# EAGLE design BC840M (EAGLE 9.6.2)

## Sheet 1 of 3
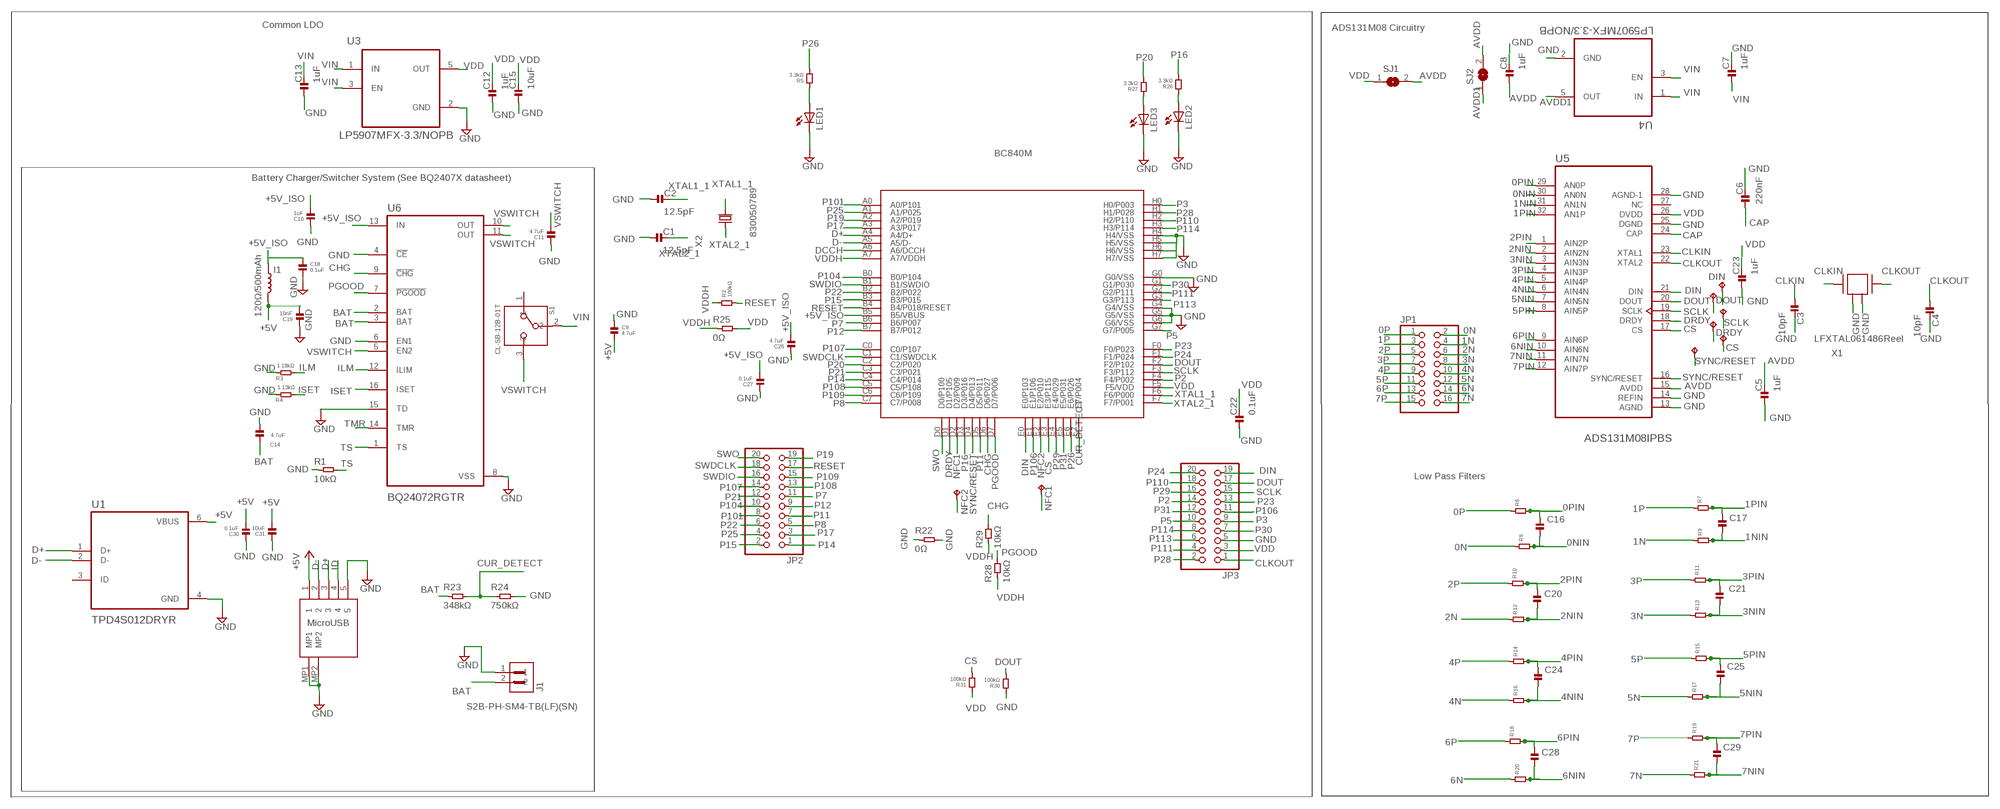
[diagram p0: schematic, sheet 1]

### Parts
C1  12.5pF  CAPACITOR.0201  [0201]
C2  12.5pF  CAPACITOR.0201  [0201]
C3  10pF  CAPACITOR.0201  [0201]
C4  10pF  CAPACITOR.0201  [0201]
C5  1uF  CAPACITOR.0201  [0201]
C6  220nF  CAPACITOR.0201  [0201]
C7  1uF  CAPACITOR.0201  [0201]
C8  1uF  CAPACITOR.0201  [0201]
C9  4.7uF  CAPACITOR.0201  [0201]
C10  1uF  CAPACITOR.0201  [0201]
C11  4.7uF  CAPACITOR.0201  [0201]
C12  1uF  CAPACITOR.0201  [0201]
C13  1uF  CAPACITOR.0201  [0201]
C14  4.7uF  CAPACITOR.0201  [0201]
C15  10uF  CAPACITOR.0402  [0402]
C16  100pF  CAPACITOR.0603  [0603]
C17  100pF  CAPACITOR.0603  [0603]
C18  0.1uF  CAPACITOR.0201  [0201]
C19  10nF  CAPACITOR.0201  [0201]
C20  100pF  CAPACITOR.0603  [0603]
C21  100pF  CAPACITOR.0603  [0603]
C22  0.1uF  CAPACITOR.0201  [0201]
C23  1uF  CAPACITOR.0201  [0201]
C24  100pF  CAPACITOR.0603  [0603]
C25  100pF  CAPACITOR.0603  [0603]
C26  4.7uF  CAPACITOR.0201  [0201]
C27  0.1uF  CAPACITOR.0201  [0201]
C28  100pF  CAPACITOR.0603  [0603]
C29  100pF  CAPACITOR.0603  [0603]
C30  0.1uF  CAPACITOR.0201  [0201]
C31  10uF  CAPACITOR.0402  [0402]
CS  TPTP07R  [TP07R]
DIN  TPTP07R  [TP07R]
DOUT  TPTP07R  [TP07R]
DRDY  TPTP07R  [TP07R]
I1  120Ω/500mAh  12NH-0402  [0402_COILCRAFT]
J1  S2B-PH-SM4-TB(LF)(SN)  [JST_S2B-PH-SM4-TB(LF)(SN)]
JP1  PINHD-2X8SMT  [2X08_SMT]
JP2  PINHD-2X10SMT  [2X10_SMT]
JP3  PINHD-2X10SMT  [2X10_SMT]
LED1  LEDCHIPLED_0603  [CHIPLED_0603]
LED2  LEDCHIPLED_0603  [CHIPLED_0603]
LED3  LEDCHIPLED_0603  [CHIPLED_0603]
NFC1  TPTP14SQ  [TP14SQ]
NFC2  TPTP14SQ  [TP14SQ]
R1  10kΩ  RESISTOR.0201  [0201]
R2  100kΩ  RESISTOR.0201  [0201]
R3  1.18kΩ  RESISTOR.0603  [0603]
R4  1.13kΩ  RESISTOR.0603  [0603]
R5  3.3kΩ  RESISTOR.0201  [0201]
R6  1MOhm  RESISTOR.0603  [0603]
R7  1MOhm  RESISTOR.0603  [0603]
R8  1MOhm  RESISTOR.0603  [0603]
R9  1MOhm  RESISTOR.0603  [0603]
R10  1MOhm  RESISTOR.0603  [0603]
R11  1MOhm  RESISTOR.0603  [0603]
R12  1MOhm  RESISTOR.0603  [0603]
R13  1MOhm  RESISTOR.0603  [0603]
R14  1MOhm  RESISTOR.0603  [0603]
R15  1MOhm  RESISTOR.0603  [0603]
R16  1MOhm  RESISTOR.0603  [0603]
R17  1MOhm  RESISTOR.0603  [0603]
R18  1MOhm  RESISTOR.0603  [0603]
R19  1MOhm  RESISTOR.0603  [0603]
R20  1MOhm  RESISTOR.0603  [0603]
R21  1MOhm  RESISTOR.0603  [0603]
R22  0Ω  RESISTOR.0805  [0805]
R23  348kΩ  RESISTOR.0603  [0603]
R24  750kΩ  RESISTOR.0603  [0603]
R25  0Ω  RESISTOR.0805  [0805]
R26  3.3kΩ  RESISTOR.0201  [0201]
R27  3.3kΩ  RESISTOR.0201  [0201]
R28  10kΩ  RESISTOR.0402  [0402]
R29  10kΩ  RESISTOR.0402  [0402]
R30  100kΩ  RESISTOR.0402  [0402]
R31  100kΩ  RESISTOR.0402  [0402]
S1  CL-SB-12B-01T  [CL-SB-12B]
SCLK  TPTP07R  [TP07R]
SJ1  SJ  [SJ]
SJ2  SJ  [SJ]
SYNC  TPTP07R  [TP07R]
U1  TPD4S012DRYR  [PSON50P145X100X60-6N]
U2  BC840M  [BC840M]
U3  LP5907MFX-3.3/NOPB  [SOT95P280X145-5N]
U4  LP5907MFX-3.3/NOPB  [SOT95P280X145-5N]
U5  ADS131M08IPBS  [QFP50P700X700X120-32N]
U6  BQ24072RGTR  [QFN50P300X300X100-17N]
U7  DX4R005JJ2R1800  [DX4R005JJ2R1800]
X1  ABM3B-8.000MHZ-B2-T  [ABM3B-8.000MHZ-B2-T]
X2  FC-12M  [FC-12M]

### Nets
0N: JP1.2 R8.1
0NIN: C16.2 R8.2 U5.30(AN0N)
0P: JP1.1 R6.1
0PIN: C16.1 R6.2 U5.29(AN0P)
1N: JP1.4 R9.1
1NIN: C17.2 R9.2 U5.31(AN1N)
1P: JP1.3 R7.1
1PIN: C17.1 R7.2 U5.32(AN1P)
2N: JP1.6 R12.1
2NIN: C20.2 R12.2 U5.2(AIN2N)
2P: JP1.5 R10.1
2PIN: C20.1 R10.2 U5.1(AIN2P)
3N: JP1.8 R13.1
3NIN: C21.2 R13.2 U5.3(AIN3N)
3P: JP1.7 R11.1
3PIN: C21.1 R11.2 U5.4(AIN3P)
4N: JP1.10 R16.1
4NIN: C24.2 R16.2 U5.6(AIN4N)
4P: JP1.9 R14.1
4PIN: C24.1 R14.2 U5.5(AIN4P)
5N: JP1.12 R17.1
5NIN: C25.2 R17.2 U5.7(AIN5N)
5P: JP1.11 R15.1
5PIN: C25.1 R15.2 U5.8(AIN5P)
6N: JP1.14 R20.1
6NIN: C28.2 R20.2 U5.10(AIN6N)
6P: JP1.13 R18.1
6PIN: C28.1 R18.2 U5.9(AIN6P)
7N: JP1.16 R21.1
7NIN: C29.2 R21.2 U5.11(AIN7N)
7P: JP1.15 R19.1
7PIN: C29.1 R19.2 U5.12(AIN7P)
+5V: C9.2 C19.2 C30.2 C31.2 I1.P$2 U1.6(VBUS) U7.1
+5V_ISO: C10.2 C18.1 C26.2 C27.2 I1.P$1 U2.B5(B5/VBUS) U6.13(IN)
AVDD: C5.2 C8.1 SJ1.2 SJ2.2 U5.15(AVDD)
AVDD1: SJ2.1 U4.5(OUT)
BAT: C14.2 J1.2 R23.1 U6.2(BAT) U6.3(BAT)
CAP: C6.1 U5.24(CAP)
CHG: R29.2 U2.D6(D6/P027) U6.9(!CHG)
CLKIN: C3.1 U5.23(XTAL1) X1.1
CLKOUT: C4.1 JP3.1 U5.22(XTAL2) X1.3
CS: CS.TP R31.1 U2.E3(E3/P115) U5.17(CS)
CUR_DETECT: R23.2 R24.1 U2.E7(E7/P004)
D+: U1.1(D+) U2.A4(A4/D+) U7.3
D-: U1.2(D-) U2.A5(A5/D-) U7.2
DCCH: U2.A6(A6/DCCH)
DIN: DIN.TP JP3.19 U2.E0(E0/P103) U5.21(DIN)
DOUT: DOUT.TP JP3.17 R30.1 U2.F2(F2/P102) U5.20(DOUT)
DRDY: DRDY.TP U2.D1(D1/P105) U5.18(DRDY)
GND: C1.1 C2.1 C3.2 C4.2 C5.1 C6.2 C7.2 C8.2 C9.1 C10.1 C11.1 C12.1 C13.1 C14.1 C15.1 C18.2 C19.1 C22.1 C23.1 C26.1 C27.1 C30.1 C31.1 J1.1 JP3.5 LED1.C LED2.C LED3.C R1.1 R3.1 R4.1 R22.1 R22.2 R24.2 R30.2 U1.4(GND) U2.G0(G0/VSS) U2.G4(G4/VSS) U2.G5(G5/VSS) U2.G6(G6/VSS) U2.H4(H4/VSS) U2.H5(H5/VSS) U2.H6(H6/VSS) U2.H7(H7/VSS) U3.2(GND) U4.2(GND) U5.13(AGND) U5.14(REFIN) U5.25(DGND) U5.28(AGND-1) U6.4(!CE) U6.6(EN1) U6.8(VSS) U6.15(TD) U7.5 U7.MP1 U7.MP2 X1.2 X1.4
ID: U7.4
ILM: R3.2 U6.12(ILIM)
ISET: R4.2 U6.16(ISET)
LED1: LED1.A R5.2
LED2: LED2.A R26.2
LED3: LED3.A R27.2
NFC1: NFC2.TP U2.D2(D2/P009)
NFC2: NFC1.TP U2.E2(E2/P010)
P2: JP3.14 U2.F4(F4/P002)
P3: JP3.9 U2.H0(H0/P003)
P5: JP3.10 U2.G7(G7/P005)
P7: JP2.11 U2.B6(B6/P007)
P8: JP2.5 U2.C7(C7/P008)
P11: JP2.7 U2.D5(D5/P011)
P12: JP2.9 U2.B7(B7/P012)
P14: JP2.1 U2.C4(C4/P014)
P15: JP2.2 U2.B3(B3/P015)
P16: R26.1 U2.D3(D3/P016)
P17: JP2.3 U2.A3(A3/P017)
P19: JP2.19 U2.A2(A2/P019)
P20: R27.1 U2.C2(C2/P020)
P21: JP2.12 U2.C3(C3/P021)
P22: JP2.6 U2.B2(B2/P022)
P23: JP3.13 U2.F0(F0/P023)
P24: JP3.20 U2.F1(F1/P024)
P25: JP2.4 U2.A1(A1/P025)
P26: R5.1 U2.E6(E6/P026)
P28: JP3.2 U2.H1(H1/P028)
P29: JP3.16 U2.E4(E4/P029)
P30: JP3.7 U2.G1(G1/P030)
P31: JP3.12 U2.E5(E5/P031)
P101: JP2.8 U2.A0(A0/P101)
P104: JP2.10 U2.B0(B0/P104)
P106: JP3.11 U2.E1(E1/P106)
P107: JP2.14 U2.C0(C0/P107)
P108: JP2.13 U2.C5(C5/P108)
P109: JP2.15 U2.C6(C6/P109)
P110: JP3.18 U2.H2(H2/P110)
P111: JP3.4 U2.G2(G2/P111)
P113: JP3.6 U2.G3(G3/P113)
P114: JP3.8 U2.H3(H3/P114)
PGOOD: R28.2 U2.D7(D7/P006) U6.7(!PGOOD)
RESET: JP2.17 R2.1 U2.B4(B4/P018/RESET)
SCLK: JP3.15 SCLK.TP U2.F3(F3/P112) U5.19(SCLK)
SWDCLK: JP2.18 U2.C1(C1/SWDCLK)
SWDIO: JP2.16 U2.B1(B1/SWDIO)
SWO: JP2.20 U2.D0(D0/P100)
SYNC/RESET: SYNC.TP U2.D4(D4/P013) U5.16(SYNC/RESET)
TMR: U6.14(TMR)
TS: R1.2 U6.1(TS)
VDD: C12.2 C15.2 C22.2 C23.2 JP3.3 R25.2 R31.2 SJ1.1 U2.F5(F5/VDD) U3.5(OUT) U5.26(DVDD)
VDDH: R2.2 R25.1 R28.1 R29.1 U2.A7(A7/VDDH)
VIN: C7.1 C13.2 S1.2 U3.1(IN) U3.3(EN) U4.1(IN) U4.3(EN)
VSWITCH: C11.2 S1.3 U6.5(EN2) U6.10(OUT) U6.11(OUT)
XTAL1_1: C2.2 U2.F6(F6/P000) X2.2
XTAL2_1: C1.2 U2.F7(F7/P001) X2.1
Unconnected: S1.1 U1.3(ID) U5.27(NC)

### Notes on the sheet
- Common LDO
- ADS131M08 Circuitry
- BC840M
- Battery Charger/Switcher System (See BQ2407X datasheet)
- 830050789
- LFXTAL061486Reel
- Low Pass Filters
- MicroUSB

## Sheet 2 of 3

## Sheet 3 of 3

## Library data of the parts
C1-C31 = standardparts:CAPACITOR
CS DIN DOUT DRDY NFC1 NFC2 SCLK SYNC = testpad:TP: Test pad
I1 = spkfncoils:12NH; MOUSER_PART: 994-0402HP-12NXGLU; PROD_ID: NDUC-15271; VALUE: 12nH
J1 = S2B-PH-SM4-TB_LF__SN_:S2B-PH-SM4-TB(LF)(SN): CONN HEADER PH SIDE 2POS 2MM SMD Check prices; AVAILABILITY: In Stock; DESCRIPTION: Connector Header Surface Mount, Right Angle 2 position 0.079 (2.00mm); MF: JST Sales; MP: S2B-PH-SM4-TB (LF)(SN); PACKAGE: None; PRICE: None
JP1 = pinhead+:PINHD-2X8: PIN HEADER
JP2 JP3 = pinhead+:PINHD-2X10: PIN HEADER
LED1-LED3 = adafruit:LED: LED
R1 R2 R4-R31 = standardparts:RESISTOR
R3 = standardparts:RESISTOR; SPICEPREFIX: R
S1 = CL-SB-12B-01T:CL-SB-12B-01T: Check prices; AVAILABILITY: In Stock; DESCRIPTION: Slide Switch SPDT Surface Mount; MF: Nidec Copal; MP: CL-SB-12B-01T; PACKAGE: None; PRICE: None
SJ1 SJ2 = jumper:SJ: SMD solder JUMPER
U1 = TPD4S012DRYR:TPD4S012DRYR: Check prices; AVAILABILITY: In Stock; DESCRIPTION: 4-channel USB ESD solution with power clamp 6-SON -40 to 85; MF: Texas Instruments; MP: TPD4S012DRYR; PACKAGE: USON-6 Texas Instruments; PRICE: None; PURCHASE-URL: https://pricing.snapeda.com/search/part/TPD4S012DRYR/?ref=eda
U2 = BC840M:BC840M: Check prices; AVAILABILITY: In Stock; DESCRIPTION: 802.15.4, Bluetooth Bluetooth v5.0, Thread, Zigbee® Transceiver Module 2.4GHz PCB Trace Surface Mount; MF: Fanstel Corp.; MP: BC840M; PACKAGE: None; PRICE: None; PURCHASE-URL: https://pricing.snapeda.com/search/part/BC840M/?ref=eda
U3 U4 = LP5907MFX-3.3_NOPB:LP5907MFX-3.3/NOPB: IC REG LINEAR 3.3V 250MA SOT23; AVAILABILITY: Unavailable; DESCRIPTION: Linear Voltage Regulator IC 1 Output 250mA SOT-23-5; MF: Texas Instruments; MP: LP5907MFX-3.3/NOPB; PACKAGE: SOT-23 Texas Instruments; PRICE: None
U5 = ADS131M08IPBS:ADS131M08IPBS: None Check prices; AVAILABILITY: Warning; DESCRIPTION: 24-bit 32-kSPS 8-channelsimultaneous-sampling delta-sigma ADC 32-TQFP -40 to 125; MF: Texas Instruments; MP: ADS131M08IPBS; PACKAGE: TQFP-32 Texas Instruments; PRICE: None; PURCHASE-URL: https://pricing.snapeda.com/search/part/ADS131M08IPBS/?ref=eda
U6 = BQ24072RGTR:BQ24072RGTR: Check prices; AVAILABILITY: In Stock; DESCRIPTION: Standalone 1-cell 1.5-A linear charger, Power Path, 4.2-V VBAT and VOUT=VBAT + 225mV 16-VQFN -40 to 85; MF: Texas Instruments; MP: BQ24072RGTR; PACKAGE: VQFN-16 Texas Instruments; PRICE: None; PURCHASE-URL: https://pricing.snapeda.com/search/part/BQ24072RGTR/?ref=eda
U7 = DX4R005JJ2R1800:DX4R005JJ2R1800: Check prices; AVAILABILITY: In Stock; DESCRIPTION: USB - micro B USB 2.0 Receptacle Connector 5 Position Surface Mount, Right Angle; Through Hole; MF: JAE Electronics; MP: DX4R005JJ2R1800; PACKAGE: None; PRICE: None
X1 = Crystals_Oscillators:ABM3B-8.000MHZ-B2-T: CRYSTAL 8.0000MHZ 18PF SMD Manufacturer's datasheet; CREATED_BY: PCBLayout.com; DIGIKEY_PART_NUMBER: 535-9720-2-ND; MANUFACTURER: Abracon LLC; MPN: ABM3B-8.000MHZ-B2-T; PACKAGE: SMD 4
X2 = crystal:FC-12M: kHz RANGE CRYSTAL UNIT

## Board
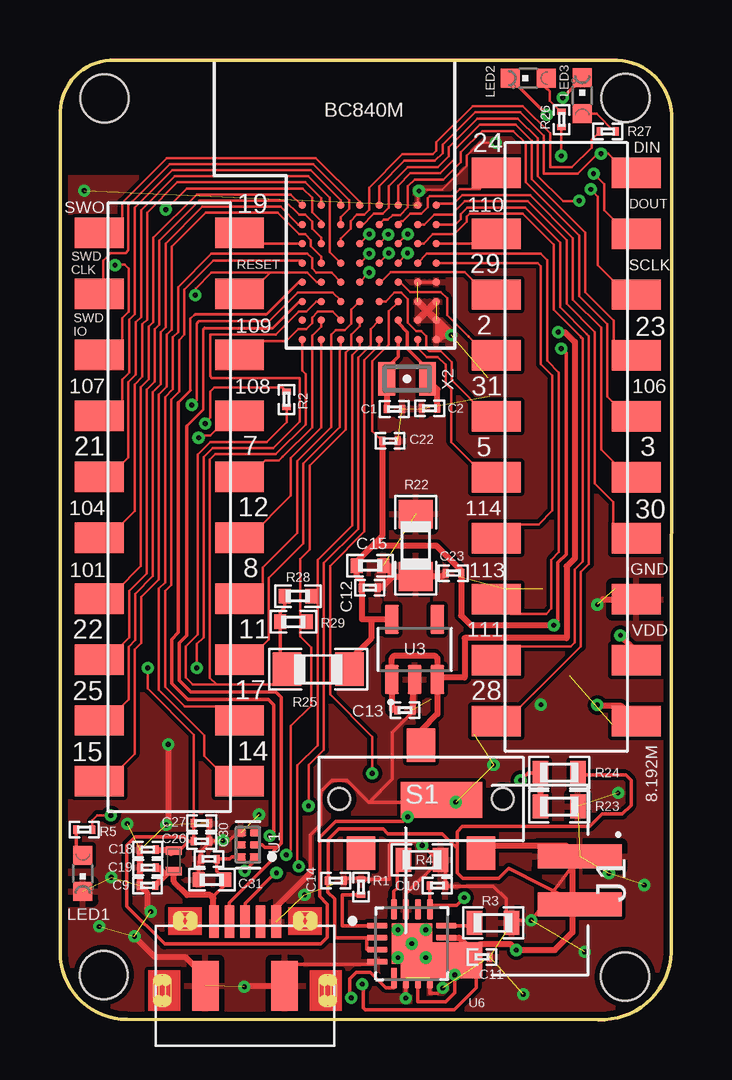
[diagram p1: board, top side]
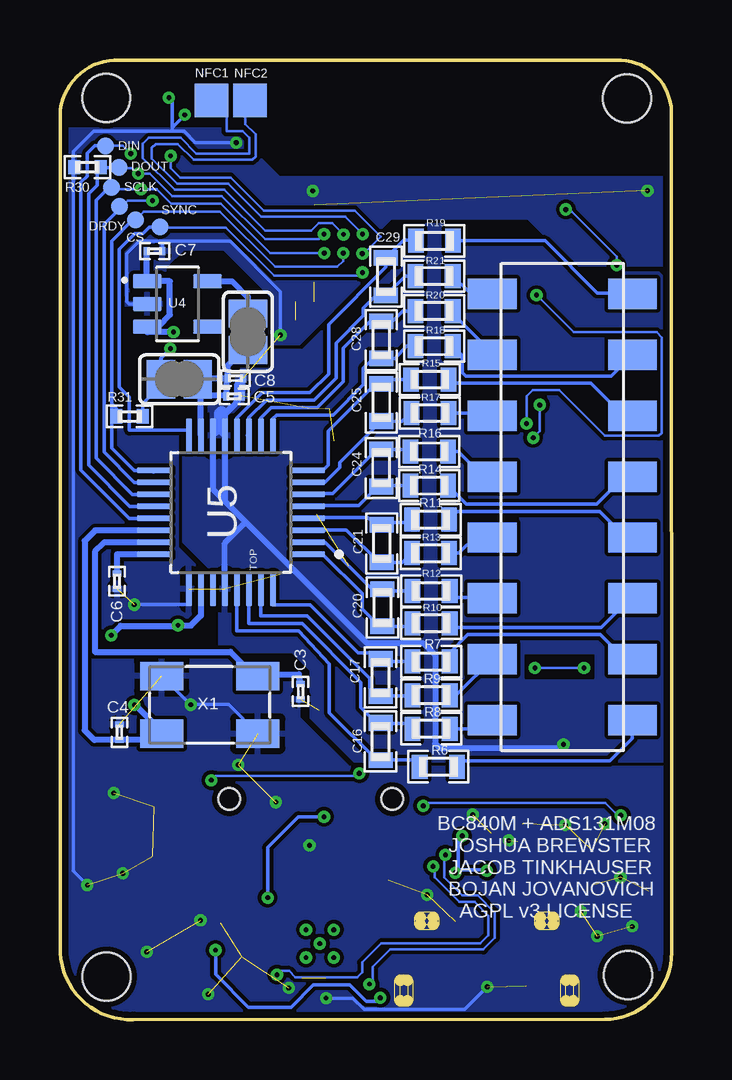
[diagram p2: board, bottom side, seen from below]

Size 25.49 x 40 mm. Coordinates in mm from the lower left corner, seen from the top.
Outline: 0,2.8 0.01,37.84 arc-90 2.3,40 23,40 arc-90 25.49,37.71 25.48,2.79 arc-90 22.43,0 2.79,0 arc-90 0,2.8
Copper layers (1*16): Top 0.035mm / dielectric 1.5mm / Bottom 0.035mm
Design rules "default *": minimum track width 4mil, minimum drill 0.2mm, track to track 6mil, track to pad 6mil, pad to pad 6mil, via to via 6mil, smd to smd 6mil, copper to edge 10mil, drill to drill 6mil, minimum pad ring 6mil, minimum via ring 6mil, stop-mask expansion 4mil, vias tented up to drill 0mil, thermal gap 10mil
Holes 2 mm at 1.86,38.4 23.56,38.42 1.82,1.86 23.54,1.79

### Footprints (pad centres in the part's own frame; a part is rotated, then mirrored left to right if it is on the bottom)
0201 = smd 0.25 x 0.35: 1 -0.325,0; 2 0.325,0
0402 = smd 0.5 x 0.6: 1 -0.55,0; 2 0.55,0
0603 = smd 0.65 x 1: 1 -0.775,0; 2 0.775,0
TP07R = smd 0.7 x 0.7: TP 0,0
0402_COILCRAFT = smd 0.356 x 0.66: P$1 -0.432,0; P$2 0.432,0
JST_S2B-PH-SM4-TB(LF)(SN) = smd 1 x 3.5: 1 1,0; 2 -1,0 | smd 1.5 x 3.4: P1 3.35,5.75; P2 -3.35,5.75
2X08_SMT = smd 1.27 x 2.032: 1 -8.89,-2.921; 2 -8.89,2.921; 3 -6.35,-2.921; 4 -6.35,2.921; 5 -3.81,-2.921; 6 -3.81,2.921; 7 -1.27,-2.921; 8 -1.27,2.921; 9 1.27,-2.921; 10 1.27,2.921; 11 3.81,-2.921; 12 3.81,2.921; 13 6.35,-2.921; 14 6.35,2.921; 15 8.89,-2.921; 16 8.89,2.921
2X10_SMT = smd 1.27 x 2.032: 1 -11.43,-2.921; 2 -11.43,2.921; 3 -8.89,-2.921; 4 -8.89,2.921; 5 -6.35,-2.921; 6 -6.35,2.921; 7 -3.81,-2.921; 8 -3.81,2.921; 9 -1.27,-2.921; 10 -1.27,2.921; 11 1.27,-2.921; 12 1.27,2.921; 13 3.81,-2.921; 14 3.81,2.921; 15 6.35,-2.921; 16 6.35,2.921; 17 8.89,-2.921; 18 8.89,2.921; 19 11.43,-2.921; 20 11.43,2.921
CHIPLED_0603 = smd 0.8 x 0.8: A 0,-0.75; C 0,0.75
TP14SQ = smd 1.4 x 1.4: TP 0,0
0805 = smd 1.2 x 1.4: 1 -1.3,0; 2 1.3,0
CL-SB-12B = smd 1.2 x 1.4: 1 -2.5,-2.25; 2 0,2.25; 3 2.5,-2.25 | hole 0.9: 3.4,0; -3.4,0
SJ = smd 1.168 x 1.6: 1 -0.762,0; 2 0.762,0
PSON50P145X100X60-6N = smd 0.42 x 0.3: 1 -0.29,0.5 | smd 0.41 x 0.3: 2 -0.295,0; 3 -0.295,-0.5; 4 0.295,-0.5; 5 0.295,0; 6 0.295,0.5
BC840M = smd 0.305 x 0.305: A0 0.66,5.966; A1 0.66,5.153; A2 0.66,4.366; A3 0.66,3.553; A4 0.66,2.765; A5 0.66,1.953; A6 0.66,1.165; A7 0.66,0.352; B0 1.448,5.966; B1 1.448,5.153; B2 1.448,4.366; B3 1.448,3.553; B4 1.448,2.765; B5 1.448,1.953; B6 1.448,1.165; B7 1.448,0.352; C0 2.261,5.966; C1 2.261,5.153; C2 2.261,4.366; C3 2.261,3.553; C4 2.261,2.765; C5 2.261,1.953; C6 2.261,1.165; C7 2.261,0.352; D0 3.048,5.966; D1 3.048,5.153; D2 3.048,4.366; D3 3.048,3.553; D4 3.048,2.765; D5 3.048,1.953; D6 3.048,1.165; D7 3.048,0.352; E0 3.861,5.966; E1 3.861,5.153; E2 3.861,4.366; E3 3.861,3.553; E4 3.861,2.765; E5 3.861,1.953; E6 3.861,1.165; E7 3.861,0.352; F0 4.648,5.966; F1 4.648,5.153; F2 4.648,4.366; F3 4.648,3.553; F4 4.648,2.765; F5 4.648,1.953; F6 4.648,1.165; F7 4.648,0.352; G0 5.461,5.966; G1 5.461,5.153; G2 5.461,4.366; G3 5.461,3.553; G4 5.461,2.765; G5 5.461,1.953; G6 5.461,1.165; G7 5.461,0.352; H0 6.248,5.966; H1 6.248,5.153; H2 6.248,4.366; H3 6.248,3.553; H4 6.248,2.765; H5 6.248,1.953; H6 6.248,1.165; H7 6.248,0.352
SOT95P280X145-5N = smd 1.21 x 0.59: 1 -1.255,0.95; 2 -1.255,0; 3 -1.255,-0.95; 4 1.255,-0.95; 5 1.255,0.95
QFP50P700X700X120-32N = smd 1.44 x 0.26: 1 -3.195,1.75; 2 -3.195,1.25; 3 -3.195,0.75; 4 -3.195,0.25; 5 -3.195,-0.25; 6 -3.195,-0.75; 7 -3.195,-1.25; 8 -3.195,-1.75; 17 3.195,-1.75; 18 3.195,-1.25; 19 3.195,-0.75; 20 3.195,-0.25; 21 3.195,0.25; 22 3.195,0.75; 23 3.195,1.25; 24 3.195,1.75 | smd 0.26 x 1.44: 9 -1.75,-3.195; 10 -1.25,-3.195; 11 -0.75,-3.195; 12 -0.25,-3.195; 13 0.25,-3.195; 14 0.75,-3.195; 15 1.25,-3.195; 16 1.75,-3.195; 25 1.75,3.195; 26 1.25,3.195; 27 0.75,3.195; 28 0.25,3.195; 29 -0.25,3.195; 30 -0.75,3.195; 31 -1.25,3.195; 32 -1.75,3.195
QFN50P300X300X100-17N = smd 0.86 x 0.26: 1 -1.435,0.75; 2 -1.435,0.25; 3 -1.435,-0.25; 4 -1.435,-0.75; 9 1.435,-0.75; 10 1.435,-0.25; 11 1.435,0.25; 12 1.435,0.75 | smd 0.26 x 0.86: 5 -0.75,-1.435; 6 -0.25,-1.435; 7 0.25,-1.435; 8 0.75,-1.435; 13 0.75,1.435; 14 0.25,1.435; 15 -0.25,1.435; 16 -0.75,1.435 | smd 1.68 x 1.68: 17 0,0 | drill 0.2 pad 0.4: 18 0,0; 19 -0.58,0.58; 20 0.58,0.58; 21 -0.58,-0.58; 22 0.58,-0.58
DX4R005JJ2R1800 = smd 1.35 x 0.4: 1 1.525,1.3; 2 1.525,0.65; 3 1.525,0; 4 1.525,-0.65; 5 1.525,-1.3 | smd 2.1 x 1.1: MP1 -1.15,1.65; MP2 -1.15,-1.65
ABM3B-8.000MHZ-B2-T = smd 1.8 x 1.2: 1 -2,-1.2; 2 2,-1.2; 3 2,1.2; 4 -2,1.2
FC-12M = smd 0.7 x 1.4: 1 -0.85,0; 2 0.85,0

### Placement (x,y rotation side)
C1  13.93,25.45 180 top
C2  15.4,25.48 0 top
C3  15.46,13.68 270 bottom
C4  23.01,11.98 90 bottom
C5  18.23,25.98 180 bottom
C6  23.11,18.27 270 bottom
C7  21.54,32.03 0 bottom
C8  18.18,26.74 0 bottom
C9  3.64,5.59 0 top
C10  15.72,5.58 180 top
C11  17.58,2.61 180 top
C12  12.91,18.01 180 top
C13  14.38,12.9 180 top
C14  11.49,5.8 180 top
C15  12.92,18.93 180 top
C16  12.13,11.59 90 bottom
C17  12.13,14.26 270 bottom
C18  3.66,7.08 180 top
C19  3.66,6.34 0 top
C20  12.05,17.17 90 bottom
C21  12.08,19.85 270 bottom
C22  13.75,24.12 180 top
C23  16.39,18.61 0 top
C24  12.11,23 90 bottom
C25  12.1,25.73 270 bottom
C26  5.9,7.43 180 top
C27  5.9,8.19 180 top
C28  12.1,28.33 90 bottom
C29  11.91,30.97 270 bottom
C30  6.21,6.7 0 top
C31  6.33,5.83 0 top
CS  22.34,33.34 0 bottom
DIN  23.59,36.42 0 bottom
DOUT  23.04,35.52 0 bottom
DRDY  23.01,33.9 0 bottom
I1  4.74,6.61 270 top
J1  21.65,5.81 90 top
JP1  4.56,21.37 90 bottom
JP2  4.55,21.36 90 top
JP3  21.09,23.87 90 top
LED1  0.95,6.09 180 top
LED2  19.5,39.25 90 top
LED3  21.76,38.52 0 top
NFC1  19.18,38.32 0 bottom
NFC2  17.57,38.32 0 bottom
R1  12.55,5.53 270 top
R2  9.44,25.85 270 top
R3  18.04,4.03 180 top
R4  15.08,6.66 180 top
R5  1.01,7.92 180 top
R6  9.73,10.54 180 bottom
R7  10.03,14.92 180 bottom
R8  10.03,12.13 180 bottom
R9  10.03,13.52 180 bottom
R10  10.03,16.52 180 bottom
R11  10.05,20.84 180 bottom
R12  10.03,17.87 180 bottom
R13  10.05,19.44 180 bottom
R14  10.1,22.26 180 bottom
R15  10.08,26.68 180 bottom
R16  10.1,23.68 180 bottom
R17  10.07,25.29 180 bottom
R18  9.9,28.07 180 bottom
R19  9.89,32.46 180 bottom
R20  9.9,29.54 180 bottom
R21  9.9,31 180 bottom
R22  14.82,19.77 90 top
R23  20.8,10.29 180 top
R24  20.8,8.88 0 top
R25  10.76,14.6 0 top
R26  20.9,37.52 90 top
R27  22.82,37.02 0 top
R28  9.92,17.65 0 top
R29  9.72,16.58 0 top
R30  24.35,35.53 180 bottom
R31  22.59,25.14 0 bottom
S1  15.04,9.19 0 top
SCLK  23.35,34.7 0 bottom
SJ1  20.52,26.7 0 bottom
SJ2  17.66,28.67 270 bottom
SYNC  21.32,33.04 0 bottom
U1  7.83,7.28 180 top
U2  9.44,27.99 0 top
U3  14.78,15.43 90 top
U4  20.6,29.83 0 bottom
U5  18.37,21.14 180 bottom
U6  14.66,3.17 0 top
U7  7.71,2.56 90 top
X1  19.25,13.12 180 bottom
X2  14.47,26.72 0 top

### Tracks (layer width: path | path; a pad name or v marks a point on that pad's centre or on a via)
0N
  Bottom 0.152: R8.1 7.83,12.13 JP1.2
0NIN
  Bottom 0.152: U5.30 17.62,16.5 15.41,16.5 12.95,14.05 12.95,13 12.31,12.37 C16.2 12.12,12.35 11.03,12.35 R8.2
0P
  Bottom 0.152: R6.1 8.95,10.78 2.59,10.78 1.64,11.73 JP1.1
0PIN
  Bottom 0.152: U5.29 18.12,16.2 15.54,16.2 14.26,14.82 14.26,12.79 12.29,10.82 C16.1 10.78,10.82 R6.2
1N
  Bottom 0.152: R9.1 9.19,13.59 8.91,13.59 JP1.4
1NIN
  Bottom 0.152: U5.31 17.12,16.83 15.19,16.83 12.58,14.23 12.58,13.81 12.26,13.48 C17.2 12.13,13.5 10.83,13.5 R9.2
1P
  Bottom 0.152: R7.1 9.25,15.29 8.49,16.05 2.98,16.05 1.95,15.02 JP1.3
1PIN
  Bottom 0.152: U5.32 16.62,17.28 15.06,17.28 13.06,15.28 12.38,15.28 C17.1 12.02,14.92 R7.2
2N
  Bottom 0.152: R12.1 8.98,17.6 7.52,17.6 JP1.6
2NIN
  Bottom 0.152: R12.2 11.97,17.87 C20.2 12.5,17.94 14.45,19.89 U5.2 | U5.2 | U5.2
2P
  Bottom 0.152: R10.1 9.08,16.35 2.94,16.35 1.73,17.56 JP1.5
2PIN
  Bottom 0.152: U5.1 14.53,19.39 12.9,17.76 12.9,17.12 12.18,16.39 C20.1 10.93,16.39 R10.2
3N
  Bottom 0.152: R13.1 8.87,19.44 8.17,20.14 7.52,20.14 JP1.8
3NIN
  Bottom 0.152: R13.2 11.22,19.05 12.06,19.05 C21.2 12.21,19.07 13.55,20.42 15.15,20.42 U5.3
3P
  Bottom 0.152: R11.1 8.94,21.18 3,21.18 1.92,20.1 JP1.7
3PIN
  Bottom 0.152: U5.4 15.13,20.93 12.67,20.93 12.36,20.62 C21.1 11.99,20.71 10.95,20.71 R11.2
4N
  Bottom 0.152: JP1.10 7.85,22.64 8.9,23.68 R16.1
4NIN
  Bottom 0.152: U5.6 15.13,21.93 14.12,21.93 12.29,23.77 C24.2 12.1,23.76 10.96,23.76 R16.2
4P
  Bottom 0.152: R14.1 8.55,21.49 3.12,21.49 1.97,22.64 JP1.9
4PIN
  Bottom 0.152: U5.5 15.13,21.43 13.04,21.43 12.25,22.22 C24.1 12.11,22.26 R14.2
5N
  Bottom 0.152: R17.1 7.59,25.29 JP1.12
5NIN
  Bottom 0.152: U5.7 15.15,22.42 14.43,22.42 13.83,23.02 13.83,23.22 C25.2 11.25,24.94 10.9,25.29 R17.2
5P
  Bottom 0.152: R15.1 9.15,26.53 3.37,26.53 2.02,25.18 JP1.11
5PIN
  Bottom 0.152: U5.8 14.54,22.89 14.31,23.12 14.31,24.54 12.35,26.5 C25.1 11.92,26.68 R15.2
6N
  Bottom 0.152: R20.1 9.08,29.49 9.08,29.39 7.49,27.81 7.49,27.73 JP1.14
6NIN
  Bottom 0.152: U5.10 17.12,25.07 16.68,25.51 14.77,25.51 13.68,26.6 13.68,27.99 12.56,29.11 C28.2 11.63,29.11 11.21,29.52 10.69,29.52 R20.2
6P
  Bottom 0.152: R18.1 8.72,27.67 8.72,26.97 8.59,26.83 2.52,26.83 JP1.13
6PIN
  Bottom 0.152: U5.9 16.62,25.05 16.46,25.2 14.11,25.2 12.85,26.46 12.85,27.15 12.44,27.56 C28.1 11.55,27.56 11.03,28.07 R18.2
7N
  Bottom 0.152: R21.1 8.43,30.3 7.52,30.3 JP1.16
7NIN
  Bottom 0.152: U5.11 17.62,25.09 16.88,25.83 14.9,25.83 13.98,26.74 13.98,28.21 12.85,29.35 12.85,29.67 12.32,30.19 C29.2 11.11,31 R21.2
  Bottom 0.254: U5.11
7P
  Bottom 0.152: R19.1 5.28,32.46 3.11,30.29 1.65,30.29 1.64,30.28 JP1.15
7PIN
  Bottom 0.152: U5.12 18.12,25.07 17.06,26.13 15.08,26.13 14.29,26.92 14.29,28.98 11.91,31.36 C29.1 11.16,32.5 10.7,32.5 R19.2
+5V
  Top 0.102: 6.43,4.11 U7.1
  Top 0.152: 4.73,6.17 I1.P$2 4.69,6.24 | 4.04,6.29 C19.2 | U1.6 7.15,6.78 7.07,6.7 C30.2 6.54,6.17 C31.2 6.88,5.62 6.39,5.13 6.39,5.06
  Top 0.254: U7.1 6.39,4.1 6.39,5.06 6.26,5.19 5.29,5.19 4.75,5.74 I1.P$2 | 4.73,6.17 4.55,6.17 C9.2 4.28,5.9 4.28,6.17 4.11,6.34 C19.2
+5V_ISO  (via drill 0.2)
  Top 0.102: U2.B5 10.69,29.94 10.26,29.51 9.95,29.51 8.99,28.55 6.27,28.55 6.26,28.54 6.26,26.82 6.33,26.75 9.98,26.75 9.98,24.93 8.88,23.82 6.36,23.82 5.99,23.45 5.99,15.94 5.7,15.65 v5.7,14.66 | v3.66,14.66 3.66,13.8 5.58,11.88 C27.2 | I1.P$1
  Top 0.152: v14.49,8.45 14.31,8.27 11.49,8.27 10.81,7.6 10.81,5.14 11.15,4.81 11.15,3.44 10.86,3.15 4.36,3.15 2.78,4.73 2.78,7.26 3.13,7.61 5.19,7.61 5.36,7.43 C26.2 | C18.1 | v16.84,5.08 16.53,4.77 15.41,4.77 U6.13 C10.2 | C26.2 5.37,7.43 4.99,7.05 I1.P$1 | C27.2 C26.2
  Top 0.254: C18.1 4.49,7.08 4.63,6.93 I1.P$1
  Bottom 0.102: v5.7,14.66 v3.66,14.66
  Bottom 0.152: v14.49,8.45 15.56,8.45 16.84,7.17 v16.84,5.08
AVDD
  Bottom 0.254: U5.15 19.62,26.02 18.6,26.02 C5.2 18.56,26.68 C8.1 | C8.1 18.5,26.74 | C8.1 18.5,27.25 17.85,27.91 SJ2.2 | SJ1.2 19.71,26.74 C8.1
AVDD1
  Bottom 0.254: U4.5 18.32,30.78 17.66,30.12 SJ2.1
BAT
  Top 0.152: J1.2 18.7,6.31 18.28,5.89 16.77,5.89 16.54,6.12 16.54,7.13 | R23.1 21.68,10.19 23.57,10.19 23.8,9.96 23.8,8.93 23.43,8.57 22.59,8.57 22.08,8.06 16.77,8.06 16.54,7.83 16.54,7.13 | 16.54,7.13 15.92,7.75 13.66,7.75 13.46,7.95 11.61,7.95 11.17,7.51 C14.2 11.17,5.31 11.45,5.03 11.45,3.42 12.77,3.42 | U6.3 13.21,2.93 12.77,2.93 12.77,3.42 | U6.2 12.77,3.42
CAP
  Bottom 0.254: U5.24 23.11,19.39 C6.1
CHG  (via drill 0.2)
  Top 0.102: U2.D6 12.48,28.9 12.13,28.55 12.13,28.02 11.91,27.8 11.91,24.59 10.41,23.09 10.41,19.6 10.01,19.2 10.01,16.63 | v9.43,6.87 9.62,7.07 9.62,12.23 10.46,13.07 10.46,15.52 10.01,15.98 10.01,16.63 | R29.2 10.22,16.63 10.01,16.63
  Top 0.152: U6.9 16.67,2.42 17.34,1.75 17.34,1.33 16.42,0.41 12.71,0.41 12.63,0.5 12.63,1.45 v12.6,1.48
  Bottom 0.102: v9.43,6.87 9.48,6.82 9.48,5.93 8.72,5.17 8.09,5.17 7.37,4.46 7.37,3.4 7.85,2.92 11.73,2.92 12.46,2.19 12.46,1.61 v12.6,1.48
CLKIN
  Bottom 0.254: U5.23 23.64,19.89 24.03,19.51 24.03,15.33 18.39,15.33 17.38,14.32 X1.1 17.17,14.39 15.53,14.39 C3.1
CLKOUT  (via drill 0.2)
  Top 0.254: v22.39,13.11 22.4,13.1 23.36,13.1 JP3.1
  Bottom 0.254: X1.3 21.65,11.92 | U5.22 24.02,20.39 24.46,19.95 24.46,12.06 24.06,11.65 C4.1 21.51,11.65 X1.3 | v22.39,13.11 22.35,13.11 21.25,12.01 X1.3
CS  (via drill 0.2 pad 0.15)
  Top 0.102: U2.E3 13.3,31.55 v13.69,31.95 | v13.69,31.95
  Bottom 0.102: v13.69,31.95 13.69,31.61 13.93,31.38 16.53,31.38 18.83,33.68 22,33.68 CS.TP
  Bottom 0.152: U5.17 22.4,22.89 23.34,23.82 23.34,25.67 | 23.34,25.67 23.34,32.46 22.45,33.34 CS.TP | R31.1 23.14,25.48 23.34,25.67
  Bottom 0.254: U5.17 21.58,22.87
CUR_DETECT  (via drill 0.2)
  Top 0.102: U2.E7 13.3,28.11 12.68,27.49 12.68,20.34 11.25,18.92 11.25,13.55 13.02,11.79 v13.02,10.26
  Top 0.152: v19.19,9.98 19.5,10.29 R23.2
  Top 0.254: R24.1 R23.2
  Bottom 0.102: v13.02,10.26 13.12,10.16 19.01,10.16 v19.19,9.98
D+  (via drill 0.2)
  Top 0.102: U2.A4 9.95,30.75 | 5.61,29.39 5.43,29.21 5.43,26.23
  Top 0.127: 9.95,30.75 8.59,29.39 5.61,29.39 | 4.94,25.73 5.43,26.23
  Top 0.152: U7.3 7.71,4.85 8.98,6.12 v9.02,6.12 | v8.73,7.66 8.9,7.83 8.9,13.12 8.67,13.35 5.32,13.35 4.66,14.01 4.66,15.85 4.94,16.13 4.94,25.73 | U1.1 8.12,6.61 v7.71,6.2
  Bottom 0.152: v8.73,7.66 8.9,7.49 8.9,6.24 v9.02,6.12 8.9,6.23 7.74,6.23 v7.71,6.2
D-
  Top 0.102: U2.A5 9.97,29.94 | 6.02,28.83 5.97,28.78 5.97,25.42
  Top 0.127: 9.97,29.94 8.87,28.83 6.02,28.83 | 5.97,25.42 5.29,24.75
  Top 0.152: U7.2 7.06,4.87 8.91,6.72 8.91,7.03 9.04,7.17 | 9.04,7.17 9.22,7.35 9.22,7.43 9.22,13.03 9.22,13.42 8.98,13.66 5.45,13.66 4.96,14.14 4.96,15.69 5.29,16.02 5.29,24.75 | 9.04,7.17 8.54,7.17 8.43,7.28 U1.2
DIN  (via drill 0.2)
  Top 0.102: U2.E0 13.3,34.74 14.35,35.8 15.61,35.8 15.94,36.12 15.94,36.47 17.29,37.82 19.18,37.82 20.17,36.84 20.17,35.27 21.58,35.27 22.41,36.1 v22.54,36.1 22.55,36.11 22.84,36.11 23.65,35.3 JP3.19
  Bottom 0.102: v22.54,36.1 22.87,36.42 DIN.TP
  Bottom 0.152: U5.21 22.61,20.89 24.62,22.9 24.62,34.9 24.35,35.17 24.35,36.12 24.05,36.42 DIN.TP
DOUT  (via drill 0.2, 0.2 pad 0.15)
  Top 0.102: U2.F2 14.31,32.58 14.32,32.58 v14.49,32.75 | v22.23,35.26 22.24,35.26 22.68,34.82 22.68,33.74 23.66,32.76 JP3.17
  Bottom 0.102: v14.49,32.75 14.7,32.53 16.93,32.53 18.74,34.34 20.82,34.34 21.74,35.26 v22.23,35.26 22.47,35.5 23.02,35.5 DOUT.TP
  Bottom 0.152: U5.20 22.58,21.39 24.3,23.11 24.3,34.43 23.94,34.78 23.94,35.3 23.73,35.52 | 23.73,35.52 DOUT.TP | R30.1 23.78,35.52 23.73,35.52
DRDY  (via drill 0.2)
  Top 0.102: U2.D1 12.54,33.08 12.57,33.08 13.07,33.59 13.44,33.59 13.7,33.85 13.7,34.74 14.5,35.54 15.74,35.54 16.19,36 16.19,36.36 17.4,37.56 19.08,37.56 19.91,36.73 19.91,35.17 20.97,34.11 21.6,34.11 v21.64,34.14
  Bottom 0.102: v21.64,34.14 22.66,34.14 22.91,33.9 DRDY.TP
  Bottom 0.152: U5.18 22.39,22.39 23.65,23.66 23.65,33.16 22.96,33.85 DRDY.TP
GND  (via drill 0.2)  (36 unrouted)
  Top 0.102: U2.G0 14.9,34.37 15.01,34.48 | 15.01,34.48 15.12,34.59 15.94,34.59 16.95,35.61 16.95,36.02 17.49,36.56 v18.15,36.56 | v14.96,34.54 15.01,34.49 15.01,34.48
  Top 0.152: U6.8 15.41,1.1 15.73,1.1 v15.95,1.32 | U7.5 9.01,4.7 | C13.1 14.7,12.82 13.85,11.96 13.85,10.02 12.88,9.06 | LED3.C 21.76,39.24 v20.95,38.43 | v20.29,37.71 LED2.C | 13.23,2.37 U6.4 13.11,2.3 9.9,2.3 9.36,1.76 U7.MP2 | U6.15 14.41,5.24 15.83,6.66 R4.1 | R4.1 16.05,6.47 C10.1 16.07,5.56 18.06,5.56 18.59,5.03 18.59,4.25 R3.1 18.93,4.13 v19.63,4.13 19.68,4.18 J1.1 | R1.1 12.5,5.9 11.92,5.9 C14.1 | R1.1 13.72,5.85 13.72,7.29 13.86,7.43 14.93,7.43 v15.09,7.26 15.11,7.26 15.71,6.66 R4.1 | R1.1 | U2.G4 U2.H4 | U6.6 14.41,0.9 v14.4,0.89 | 10.43,6.12 10.43,7.71 10.86,8.14 10.86,9.52 11.32,9.97 11.97,9.97 12.88,9.06 | 12.88,9.06 v16.49,9.06 | C31.1 5.78,6.59 C30.1 5.89,7.03 6.32,7.46 v6.79,7.46 7.06,7.46 7.38,7.79 U1.4 | 6.42,7.43 C26.1 C27.1
  Top 0.254: U7.MP1 6.06,1.78 5.23,2.6 3.96,2.6 v3.1,3.47 | U3.2 14.7,14.1 14.7,13.87 | 14.7,13.87 C13.1 | 14.7,13.87 | 9.01,4.7 10.43,6.12 | v4.51,11.48 4.51,8.29 4.43,8.21 v4.43,8.12 | v7.68,1.37 7.73,1.41 U7.MP2 | C18.2 C19.1 3.32,6.32 C9.1 3.64,5.28 3.64,4.65 v3.79,4.5 | 13.87,18.47 13.4,18.01 C12.1 | 13.87,18.47 13.75,18.47 13.75,18.86 13.68,18.93 C15.1 | 13.87,18.47 R22.1 15.92,18.47 C23.1 | v22.39,17.29 22.62,17.52 JP3.5
  Top 0.305: U2.G5 U2.H6 | U2.G6 U2.H5 | U2.H6 16.3,28.55 v16.3,28.53 | v16.3,28.53 v16.31,28.53 15.93,28.53 15.79,28.38 | v16.3,28.53 | 15.79,28.38 15.75,28.34 U2.H7 | U2.H6 15.79,29.05 15.79,28.38
  Bottom 0.102: C8.2 17.84,26.73
  Bottom 0.152: U4.2 22.6,29.83 22.71,29.94 22.71,31.94 22.19,32.45 21.2,32.45 | v18.15,36.56 19.85,36.56 20.32,37.03 20.81,37.03 | 24.93,35.57 24.93,36.19 24.09,37.03 20.81,37.03 | 24.93,35.57 24.93,6.19 v24.35,5.61 | v20.29,37.71 v20.29,37.7 20.61,37.38 20.81,37.19 | v20.95,38.43 20.81,38.29 20.81,37.19 | 20.81,37.19 20.81,37.03 | 21.2,32.45 21.22,32.43 C7.2 | v16.3,28.53 16.3,30.35 18.4,32.45 21.2,32.45 | 18.7,25.3 18.77,25.22 | 18.56,25.33 18.7,25.19 18.7,25.3 | 18.7,25.45 18.7,25.3 | R30.2 24.93,35.57 | U5.25 20.12,17.29 v22.39,17.29 | X1.4 18.46,13.13 v20.04,13.13 20.06,13.13 X1.2 | v14.4,0.89 13.28,0.89 12.82,0.43 8.62,0.43 v7.68,1.37
  Bottom 0.254: 18.32,25.53 18.36,25.53 18.56,25.33 | 18.77,25.22 18.77,24.5 U5.13 | 18.7,25.45 18.81,25.45 18.95,25.3 18.95,24.5 U5.14 19.12,22.11 18.62,21.61 | 18.15,25.69 18.1,25.74 18.1,26.49 C8.2 17.91,26.68 C5.1 18.15,25.74 18.15,25.69 | 18.62,21.61 17.74,20.74 | 17.74,20.74 12.7,15.7 10.36,15.7 9.86,15.19 9.86,11.51 9.67,11.33 4.66,11.33 v4.51,11.48 | U5.28 18.62,19.86 17.74,20.74 | U5.13 18.62,21.61 | 18.15,25.69 18.32,25.53 | 18.32,25.53 18.62,25.23 U5.13
  other vias: 2.13,5.93 18.06,10.62 21.87,2.82 22.87,6.09 1.01,34.55 23.25,9.44 2.8,8.17 19.31,1.05 8.29,8.54 1.64,3.88 10.19,5.2
  pour Top: 1.46,-0.28 -0.01,1.19 -0.01,35.1 16.75,35.1 16.75,36.07 17.75,37.07 25.64,37.07 25.64,1.36 24,-0.28
  pour Bottom: -0.29,30.28 0.55,31.11 4.1,31.11 6.13,33.14 11.47,33.14 12.47,32.14 12.47,30.78 15.36,27.88 16.89,27.88 16.89,30.03 18.7,31.84 20.24,31.84 20.82,31.25 20.82,28.53 20.32,28.03 20.32,19.9 18.83,18.41 18.83,15.35 15.82,15.35 15.02,14.55 15.02,12.57 13.24,10.78 -0.29,10.78
  pour Bottom: 0.04,31.44 4.01,31.44 5.97,33.41 11.71,33.41 12.68,32.44 12.68,31.03 15.52,28.19 16.67,28.19 16.67,30.14 18.65,32.13 20.36,32.13 21.12,31.36 21.12,28.38 20.6,27.87 20.6,19.67 19.09,18.16 19.09,15.37 18.76,15.04 15.97,15.04 15.53,14.6 15.53,12.57 13.47,10.5 -0.23,10.5 -0.23,1.48 1.55,-0.3 24.02,-0.3 25.69,1.37 25.69,37.12 18.39,37.12 16.36,35.1 0.04,35.1
  cutout Bottom: 3.28,15.18 3.28,14.24 6.07,14.24 6.07,15.18
ILM
  Top 0.152: U6.12 17.29,3.92 R3.2
ISET
  Top 0.152: U6.16 13.91,5.34 14.05,5.48 14.05,6.41 R4.2
LED1
  Top 0.102: R5.2
  Top 0.152: R5.2 0.68,7.11 LED1.A
LED2
  Top 0.102: LED2.A 20.25,39.24 20.25,38.85 20.4,38.69 20.4,38.31 20.86,37.84 R26.2
LED3
  Top 0.102: R27.2 23.1,37.02 22.36,37.77 LED3.A
NFC1  (via drill 0.2)
  Top 0.102: U2.D2 v12.88,32.75
  Bottom 0.102: v12.88,32.75 13.61,33.47 17.11,33.47 18.48,34.84 20.61,34.84 21.66,35.89 21.66,36.34 21.5,36.5 20.58,36.5 19.91,35.84 17.47,35.84 17.34,35.97 17.34,36.9 17.78,37.33 17.78,38.11 NFC2.TP
NFC2  (via drill 0.2)
  Top 0.102: U2.E2 v13.67,32.73
  Bottom 0.102: NFC1.TP 18.55,37.68 18.55,37.03 17.88,37.03 17.6,36.75 17.6,36.11 17.61,36.1 19.81,36.1 20.46,36.75 21.79,36.75 22.03,36.51 22.03,35.91 20.71,34.59 18.64,34.59 16.94,32.9 15.02,32.9 14.71,33.21 14.15,33.21 v13.67,32.73
P2  (1 unrouted)
  Top 0.102: U2.F4 14.17,30.75 14.59,30.33 15.86,30.33 16.13,30.07 16.13,29.37 17,28.5 | JP3.14 17.82,27.68 17.03,28.47
P3
  Top 0.102: U2.H0 15.75,34.02 16.42,34.02 16.76,34.36 19.59,34.36 21.37,32.58 21.37,30.02 22.54,28.84 22.54,23.77 23.38,22.93 23.69,22.93 JP3.9
P5
  Top 0.102: U2.G7 14.9,27.99 15.27,27.62 15.75,27.62 16.07,27.3 16.07,26.51 16.3,26.28 16.3,24.08 17.79,22.6 JP3.10
P7
  Top 0.102: U2.B6 10.88,28.89 10.5,28.51 10.5,24.69 9.29,23.48 9.12,23.31 8.54,23.31 7.87,22.63 JP2.11
P8
  Top 0.102: U2.C7 11.7,27.95 11.66,27.91 11.66,24.7 10.14,23.18 10.14,19.85 8.69,18.41 8.69,15.85 7.86,15.01 JP2.5
P11
  Top 0.102: U2.D5 12.46,29.94 12.13,29.6 12.13,29.01 11.86,28.74 11.49,28.74 11.29,28.55 11.29,24.7 9.88,23.28 9.88,20.28 8.44,18.84 8.44,18.17 7.82,17.55 JP2.7
P12
  Top 0.102: U2.B7 10.89,24.68 9.62,23.41 9.62,21.84 7.88,20.09 JP2.9
P14
  Top 0.102: U2.C4 11.32,31.13 10.69,31.13 10.5,31.31 10.5,31.74 10.31,31.93 6.31,31.93 4.92,30.54 4.92,28.65 4.71,28.44 4.71,26.28 4.38,25.95 4.38,18.23 4.12,17.97 4.12,13.74 6.02,11.84 6.02,11 7.09,9.93 JP2.1
P15
  Top 0.102: U2.B3 10.88,31.81 10.45,32.24 10.45,32.5 10.22,32.74 9.98,32.74 9.08,33.63 6.06,33.63 4.66,32.22 4.66,28.76 4.45,28.55 4.45,26.38 4.13,26.05 4.13,18.34 3.39,17.61 3.39,15.71 3.11,15.43 3.11,11.07 1.97,9.93 JP2.2
P16  (via drill 0.2, 0.2 pad 0.15)
  Top 0.102: U2.D3 12.51,31.54 v12.89,31.92 v12.89,31.93 | R26.1 20.88,37.17 v20.88,36
  Bottom 0.102: v12.89,31.93 12.84,31.93 12.13,32.64 13.21,33.73 17,33.73 18.38,35.1 20.49,35.1 20.88,35.5 v20.88,36
P17
  Top 0.102: U2.A3 10.01,31.63 6.38,31.63 5.18,30.43 5.18,28.55 4.96,28.33 4.96,26.17 4.63,25.84 4.63,18.12 4.38,17.87 4.38,13.87 5.2,13.05 6.52,13.05 7.17,12.41 7.41,12.41 JP2.3
P19
  Top 0.102: U2.A2 9.19,32.35 | 9.19,32.35 9.18,32.35 | 9.19,32.35 7.92,32.35 JP2.19
P20
  Top 0.102: U2.C2 11.7,32.55 12.11,32.96 12.11,33.29 12.37,33.55 12.67,33.55 12.88,33.77 12.88,34.69 14.27,36.07 15.53,36.07 15.68,36.23 15.68,36.57 17.19,38.07 19.29,38.07 20.42,36.94 20.42,35.53 21.33,35.53 22.15,36.35 22.15,36.67 R27.1
P21
  Top 0.102: U2.C3 11.24,32 11.24,34.25 10.34,35.15 4.78,35.15 3.38,33.75 3.38,29.29 3.16,29.07 3.16,26.88 2.85,26.58 2.85,23.43 2.05,22.63 JP2.12
P22
  Top 0.102: U2.B2 10.88,32.6 10.5,32.98 10.5,33.27 10.22,33.55 9.96,33.55 9.37,34.14 5.81,34.14 4.14,32.47 4.14,28.97 3.95,28.77 3.95,26.59 3.62,26.27 3.62,18.6 2.88,17.87 2.88,15.92 1.97,15.01 JP2.6
P23
  Top 0.102: U2.F0 14.08,34.77 14.6,35.28 15.85,35.28 16.45,35.88 16.45,36.26 17.49,37.3 18.99,37.3 19.65,36.63 19.65,35.04 21.88,32.81 21.88,30.34 23.07,29.14 23.07,28.23 23.63,27.68 JP3.13
P24
  Top 0.102: U2.F1 14.23,33.28 14.28,33.28 14.59,33.6 15.04,33.6 15.31,33.86 15.31,34.24 15.41,34.33 16.37,34.33 16.65,34.61 17.49,34.61 JP3.20
P25
  Top 0.102: U2.A1 9.94,33.14 9.19,33.88 5.93,33.88 4.4,32.35 4.4,28.86 4.2,28.66 4.2,26.49 3.87,26.16 3.87,18.48 3.14,17.75 3.14,15.82 2.86,15.54 2.86,13.35 1.98,12.47 JP2.4
P26  (via drill 0.2)
  Top 0.102: U2.E6 12.94,28.79 12.94,28.11 12.42,27.59 12.42,20.46 10.99,19.03 10.99,11.25 10.36,10.61 v10.36,8.91 | v2.12,8.51 1.55,8.51 1.33,8.3 R5.1
  Bottom 0.102: v10.36,8.91 10.24,9.03 2.77,9.03 2.25,8.51 v2.12,8.51
P28
  Top 0.102: U2.H1 15.76,33.14 16.47,33.14 16.7,33.37 16.7,33.58 16.97,33.85 19.38,33.85 20.84,32.39 20.84,29.7 21.96,28.58 22.03,28.5 22.03,18.98 21.71,18.65 21.71,15.55 18.6,12.44 JP3.2
P29
  Top 0.102: U2.E4 13.37,30.75 13.78,31.16 16.86,31.16 17.81,30.22 JP3.16
P30
  Top 0.102: U2.G1 15.18,33.14 15.59,33.55 16.45,33.55 16.45,33.69 16.86,34.11 19.48,34.11 21.11,32.49 21.11,29.85 22.29,28.67 22.29,22.34 23.05,21.58 23.05,20.7 23.68,20.06 JP3.7
P31
  Top 0.102: U2.E5 13.58,29.94 13.94,30.3 14.23,30.3 14.49,30.03 14.49,29.05 14.85,28.69 15.04,28.69 15.25,28.48 15.25,28.01 15.39,27.87 15.86,27.87 16.32,27.41 16.32,26.65 17.83,25.14 JP3.12
P101
  Top 0.102: U2.A0 10.06,33.95 9.62,34.39 5.69,34.39 3.89,32.59 3.89,29.08 3.69,28.88 3.69,26.7 3.36,26.37 3.36,18.9 2.36,17.9 1.98,17.9 JP2.8
P104
  Top 0.102: U2.B0 10.88,34.24 10.22,34.9 4.89,34.9 3.63,33.64 3.63,29.18 3.44,28.99 3.44,26.8 3.11,26.47 3.11,21.21 1.99,20.09 JP2.10
P106
  Top 0.102: U2.E1 13.5,33.34 13.67,33.34 13.86,33.54 14.17,33.54 14.49,33.86 14.49,34.74 14.77,35.02 15.98,35.02 16.7,35.74 16.7,36.15 17.59,37.04 18.89,37.04 19.4,36.53 19.4,34.92 21.63,32.69 21.63,30.16 22.8,28.99 22.8,25.98 23.64,25.14 JP3.11
P107
  Top 0.102: U2.C0 11.7,34.16 10.45,35.41 4.68,35.41 3.12,33.85 3.12,29.41 2.89,29.18 2.89,26.98 2.59,26.68 2.59,25.76 2,25.17 JP2.14
P108  (via drill 0.2 pad 0.15)
  Top 0.102: U2.C5 11.7,29.98 11.37,30.31 9.91,30.31 8.71,29.11 5.79,29.11 5.7,29.02 5.7,25.83 v5.5,25.62 | JP2.13 7.08,25.17 6.25,24.34 5.86,24.34 v5.77,24.25
  Bottom 0.102: v5.77,24.25 5.49,24.53 v5.49,25.62 v5.5,25.62
P109
  Top 0.102: U2.C6 11.7,29.17 11.36,29.51 10.74,29.51 10.5,29.27 10.5,29.03 10.25,28.78 9.94,28.78 9.44,28.27 8.04,28.27 JP2.15
P110
  Top 0.102: U2.H2 15.74,32.35 15.75,32.35 16.94,32.35 17.76,32.35 JP3.18
P111
  Top 0.102: U2.G2 15.15,32.35 15.54,32.74 16.43,32.74 16.95,33.26 16.95,33.48 17.07,33.6 19.27,33.6 20.58,32.29 20.58,29.6 21.7,28.47 21.7,28.46 21.78,28.38 21.78,19.09 21.45,18.76 21.45,15.73 21.29,15.56 18.76,15.56 JP3.4
P113
  Top 0.102: U2.G3 15.28,31.92 20.04,31.92 20.3,31.65 20.3,27.46 20.79,26.98 20.79,19.48 20.47,19.16 20.47,17.13 20.25,16.91 18.78,16.91 JP3.6
P114
  Top 0.102: U2.H3 19.91,31.54 20.04,31.41 20.04,27.32 20.52,26.84 20.52,21.21 19.95,20.64 18.76,20.64 JP3.8
PGOOD  (via drill 0.2)
  Top 0.102: U2.D7 12.48,28.02 12.17,27.7 12.17,20.59 10.73,19.16 10.73,17.69 | v9.94,6.39 9.89,6.45 9.89,10.59 10.73,11.44 10.73,17.69 | R28.2 10.5,17.69 10.73,17.69
  Top 0.152: U6.7 14.91,0.74 16.07,0.74 16.45,1.12 v16.45,1.87
  Bottom 0.102: v9.94,6.39 9.88,6.32 9.88,5.93 8.85,4.9 8.2,4.9 7.64,4.33 7.64,3.52 7.98,3.18 12.1,3.18 12.9,2.38 12.9,1.96 13.1,1.77 15.68,1.77 15.94,2.03 16.45,2.03 v16.45,1.87
RESET  (via drill 0.2)
  Top 0.102: U2.B4 10.7,30.75 10.31,31.14 8.77,31.14 | 8.77,31.14 6.31,31.14 5.65,30.48 v5.65,30.21 v5.63,30.2 | v6.05,24.85 6.05,24.89 6.25,25.09 6.25,26.17 6.42,26.34 9.28,26.34 R2.1 | 8.77,31.14 8.14,30.51 7.73,30.51 JP2.17
  Bottom 0.102: v5.63,30.2 5.62,30.2 4.08,28.65 0.63,28.65 0.42,28.44 0.42,24.46 0.54,24.34 2.78,24.34 4.69,26.25 5.79,26.25 6.05,25.99 v6.05,24.85
SCLK  (via drill 0.2, 0.2 pad 0.15)
  Top 0.102: v14.48,31.95 14.08,31.56 U2.F3 | v22.11,34.61 22.41,34.31 22.41,31.45 23.65,30.22 JP3.15
  Bottom 0.102: v14.48,31.95 16.73,31.95 18.79,34.02 20.86,34.02 21.46,34.61 v22.11,34.61 23.26,34.61 SCLK.TP
  Bottom 0.152: U5.19 22.47,21.89 23.98,23.4 23.98,34.15 23.43,34.7 SCLK.TP
SWDCLK
  Top 0.102: U2.C1 11.7,33.45 12.05,33.8 12.05,34.17 10.56,35.66 4.57,35.66 3.01,34.1 | 3.01,34.1 2.97,34.06 | 3.01,34.1 2.85,33.94 2.85,32.07 2.73,31.95 2.12,31.95 1.8,31.64 1.8,30.42 JP2.18
SWDIO  (via drill 0.2 pad 0.15)
  Top 0.102: U2.B1 10.88,33.29 10.5,33.67 10.5,34.26 10.12,34.65 5.29,34.65 v4.41,33.77 | v2.29,31.45 2.32,31.47 2.69,31.47 2.87,31.3 2.87,29.51 2.6,29.25 2.6,28.31 2,27.71 JP2.16
  Bottom 0.102: v4.41,33.77 4.33,33.69 4.17,33.69 2.29,31.81 v2.29,31.45
SWO
  Top 0.102: U2.D0 12.48,34.1 10.67,35.92 4.44,35.92 2.59,34.06 2.59,33.31 2.08,32.79 JP2.20
SYNC/RESET  (via drill 0.2 pad 0.15)
  Top 0.102: U2.D4 12.85,31.12 12.87,31.12 12.87,31.13 v12.88,31.15
  Bottom 0.102: v12.88,31.15 13.02,31.01 16.56,31.01 18.58,33.02 21.31,33.02 SYNC.TP
  Bottom 0.152: U5.16 20.12,24.57 22.59,24.57 22.59,25.96 23.01,26.38 23.01,32.11 22.37,32.75 22.05,32.75 21.77,33.04 SYNC.TP
TS
  Top 0.152: U6.1 11.77,3.92 11.77,5.2 R1.2
VDD  (via drill 0.2)
  Top 0.102: 14.08,29.92 13.7,29.53 13.7,28.14 13.02,27.45 13.02,24.53 C22.2
  Top 0.152: 14.08,29.92 U2.F5 | v20.57,16.44 20.75,16.62 20.75,19.05 21.08,19.38 21.08,27.78 v20.89,27.97
  Top 0.254: 12.96,16.68 12.96,15.89 12.06,14.99 R25.2 | 13.8,16.71 U3.5 12.96,16.68 | C22.2 13.42,20.15 13.02,19.74 | C23.2 | C23.2 16.71,16.84 17.14,16.42 20.55,16.42 v20.57,16.44 | 13.02,19.74 12.37,19.1 C15.2 12.37,18.5 12.58,18.3 12.58,18.01 C12.2 12.57,18 12.57,16.68 12.96,16.68 | C23.2 16.71,18.72 15.69,19.74 13.02,19.74 | JP3.3 24.02,15.36 v23.35,16.02
  Bottom 0.152: SJ1.1 21.28,27.58 v20.89,27.97 21.28,27.58 21.28,26.44 22.04,25.68 R31.2
  Bottom 0.254: U5.26 19.62,16.84 20.04,16.42 20.55,16.42 v20.57,16.44 20.57,16.41 22.96,16.41 v23.35,16.02
VDDH
  Top 0.102: R2.2 9.44,24.91 8.61,24.08 6.26,24.08 5.73,23.56 5.73,16.05 5.24,15.56 5.24,14.27 5.54,13.98 6.52,13.98 | 6.52,13.98 6.25,14.25 6.25,23.35 6.47,23.57 9,23.57 10.24,24.81 10.24,26.92 10.1,27.06 U2.A7 | 6.52,13.98 8.84,13.98 R25.1
  Top 0.152: R28.1 9.37,17.18 9.17,16.99 R29.1 9.17,15.24 9.46,14.95 R25.1
VIN  (via drill 0.2)
  Top 0.254: U3.3 15.82,14.26 16.85,14.25 16.85,15.9 21.11,15.9 21.11,18.89 21.45,19.23 21.45,28.24 21.04,28.65 v20.76,28.65 | C13.2 13.83,12.9 U3.1 13.83,15.07 13.94,15.18 15.61,15.18 15.73,15.06 U3.3 | U3.3 15.73,12.74 15.04,12.05 S1.2 15.04,11.07
  Bottom 0.254: C7.1 21.87,30.8 U4.1 20.91,30.78 20.91,29.38 21.37,28.92 21.81,28.92 U4.3 21.85,28.65 v20.76,28.65
VSWITCH  (via drill 0.2)
  Top 0.152: v12.14,0.91 12.14,0.99 12.08,1.05 12.08,1.7 12.35,1.97 12.94,1.97 13.57,1.33 13.91,1.33 U6.5
  Top 0.254: S1.3 17.84,7.24 21.08,7.24 21.35,6.97 21.35,3.63 20.62,2.9 v19.01,2.9 18.76,3.15 17.51,3.15 17.26,2.9 C11.2 17.26,2.79 16.63,3.42 U6.11 | U6.10 17.05,2.92
  Bottom 0.152: v19.01,2.9 19.01,1.88 17.65,0.52 15.86,0.52 14.93,1.45 13.41,1.45 12.73,0.77 12.28,0.77 v12.14,0.91
XTAL1_1
  Top 0.152: U2.F6 14.08,29.04 14.47,28.66 14.47,27.97 15.32,27.12 X2.2
  Top 0.254: X2.2 15.3,26.7 15.73,26.27 C2.2
XTAL2_1
  Top 0.152: U2.F7 14.08,27.64 13.62,27.17 X2.1
  Top 0.254: X2.1 13.6,26.7 C1.2

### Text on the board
tPlace: BC840M | 24 | DIN | SWO | 19 | 110 | DOUT | RESET | SCLK | SWD / CLK | 29 | SWD / IO | 109 | 2 | 23 | 107 | 108 | 31 | 106 | 21 | 7 | 5 | 3 | 104 | 12 | 114 | 30 | 101 | 8 | 113 | GND | 22 | 11 | 111 | VDD | 25 | 17 | 28 | 15 | 14 | 8.192M
bPlace: TOP | BC840M + ADS131M08 / JOSHUA BREWSTER / JACOB TINKHAUSER / BOJAN JOVANOVICH / AGPL v3 LICENSE
tNames: R2 | S1
Measures: Notes: / - Minimize space without jeopardizing grounding for the external ADC / i.e. be keen with ground plane traces and electron flow. / - Break out all unused programmable pins plus ADC inputs. / ADC inputs may have to be a (CHEAP) SMT connector backside to minimize possible interference from the radio, / but let's just break them out first and test. Let's still ID a 16-20 pin connector.
Document: SWO | SWDCLK | RESET | SWDIO | GND | VDD
bDocu: GND | VDD | 8.192MHz

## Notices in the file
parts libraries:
spkfncoils: Licensing: Creative Commons ShareAlike 4.0 International - https://creativecommons.org/licenses/by-sa/4.0
